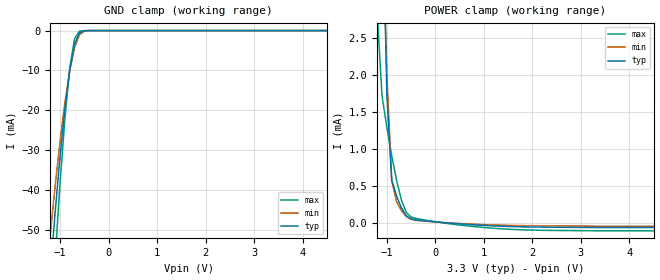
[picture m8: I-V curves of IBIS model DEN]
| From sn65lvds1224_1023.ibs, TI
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|   Model DEN
| Developed by Ayah Elkhordagy
[Model]   DEN
Model_type   Input
Polarity   Non-Inverting
| Vinl and vih from datasheet
Vinl = 0.8
Vinh = 2.0
| ccomp values are extracted by ICX.
C_comp   0.859pF   0.832pF   0.88pF
[Temperature Range]   27   85   -40
[Voltage Range]   3.3V   3.0V   3.6V
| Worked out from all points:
|   GND clamp passes 1 mA (typ) near -0.62 V on its own axis
|   POWER clamp passes 1 mA (typ) near -0.94 V on its own axis
[GND_clamp]
| voltage   I(typ)   I(min)   I(max)
-3.3V     -471.9mA   -392.6mA   -586.6mA
-1.2V     -60.89mA   -51.24mA   -77.81mA
-1.1V     -45.7mA    -39.03mA   -57.39mA
-1V       -31.87mA   -27.96mA   -38.64mA
-900mV    -19.8mA    -18.23mA   -22.27mA
-800mV    -9.998mA   -10.14mA   -9.442mA
-700mV    -3.379mA   -4.239mA   -2.07mA
-600mV    -572.3uA   -1.09mA    -165.4uA
-500mV    -52uA      -161.7uA   -7.6uA
-300mV    -1.57uA    -2.7uA     -1.5uA
6.6V      0A         0A         0A
[POWER_clamp]
| voltage   I(typ)   I(min)   I(max)
-3.3V     119.9mA    83.74mA    140.6mA
-1.2V     8.681mA    6.762mA    2.855mA
-1.1V     4.909mA    4.211mA    1.722mA
-1V       1.738mA    2.007mA    1.296mA
-900mV    580.2uA    574.1uA    911.7uA
-800mV    363.6uA    287.6uA    577uA
-700mV    201.8uA    168.1uA    309.8uA
-600mV    98.92uA    87.89uA    141.4uA
-500mV    55.71uA    48.31uA    79.73uA
500mV     -13.11uA   -7.661uA   -28.24uA
1.7V      -52.26uA   -35.39uA   -91.19uA
6.6V      -62.2uA    -45.38uA   -106.2uA
